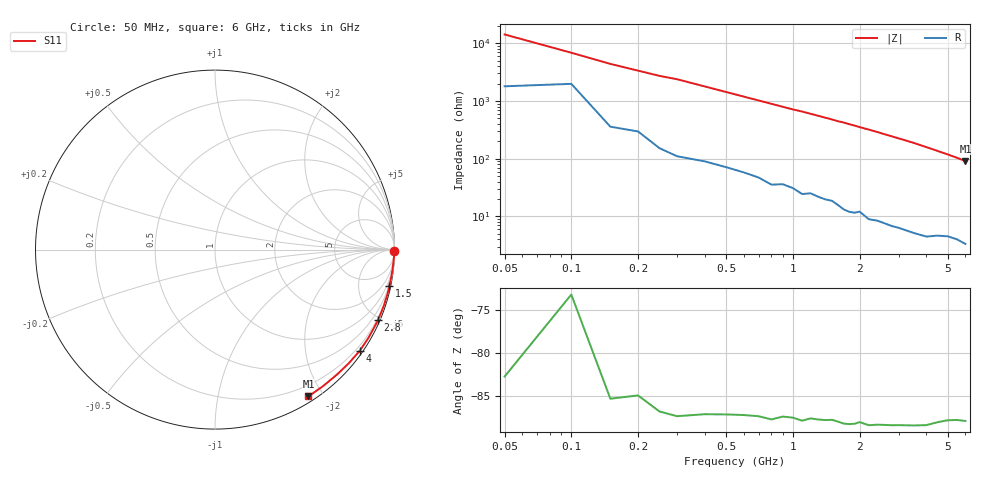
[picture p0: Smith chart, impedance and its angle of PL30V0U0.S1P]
! Infineon Technologies  Discrete & RF Semiconductors
! BAR 64-04W /-05W /-06W
! Si PIN Diode in SOT323
! VR = 30 V
! S-Parameters:  October  2008
# GHz  S  MA  R  50
!  f  S11
! GHz  MAG  ANG
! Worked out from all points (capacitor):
!   34 points, 50 MHz to 6 GHz, reference 50 ohm
!   read as one part to ground: C = 242 fF near 50 MHz
!   lowest |Z| = 91.1 ohm at 6 GHz (marker M1)
!   S11 on the Smith chart (normalised r, x): 50 MHz: open; 1.5 GHz: 0.37, -9.58; 2.8 GHz: 0.14, -4.87; 4 GHz: 0.09, -3.18; 6 GHz: 0.07, -1.82
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0.05  0.9991 -0.4
0.1  0.9958 -0.8
0.15  0.9981 -1.3
0.2  0.9974 -1.7
0.25  0.998 -2.1
0.3  0.9981 -2.4
0.8  0.9956 -6.4
1  0.994 -8.0
1.1  0.9944 -8.7
1.2  0.9931 -9.5
1.4  0.9926 -11.1
1.5  0.992 -11.9
1.6  0.9922 -12.8
1.7  0.9928 -13.5
1.8  0.9925 -14.4
1.9  0.9919 -15.2
2  0.9905 -16.1
2.2  0.9915 -17.8
2.4  0.9903 -19.5
2.6  0.9896 -21.4
2.8  0.989 -23.2
3  0.9881 -25.0
3.5  0.9865 -29.7
4  0.984 -34.9
4.5  0.9781 -40.3
5  0.973 -45.7
5.5  0.9703 -51.4
6  0.9695 -57.5
